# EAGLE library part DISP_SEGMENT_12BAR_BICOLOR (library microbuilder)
12-Bar Bi-Color LED Segment Displays: Row = Cathode 30.2 x 10.1mm Bi-Color 12 LED Bar Graph, 5.0 x 1.74mm Square LEDs - BL-AR12Z3010
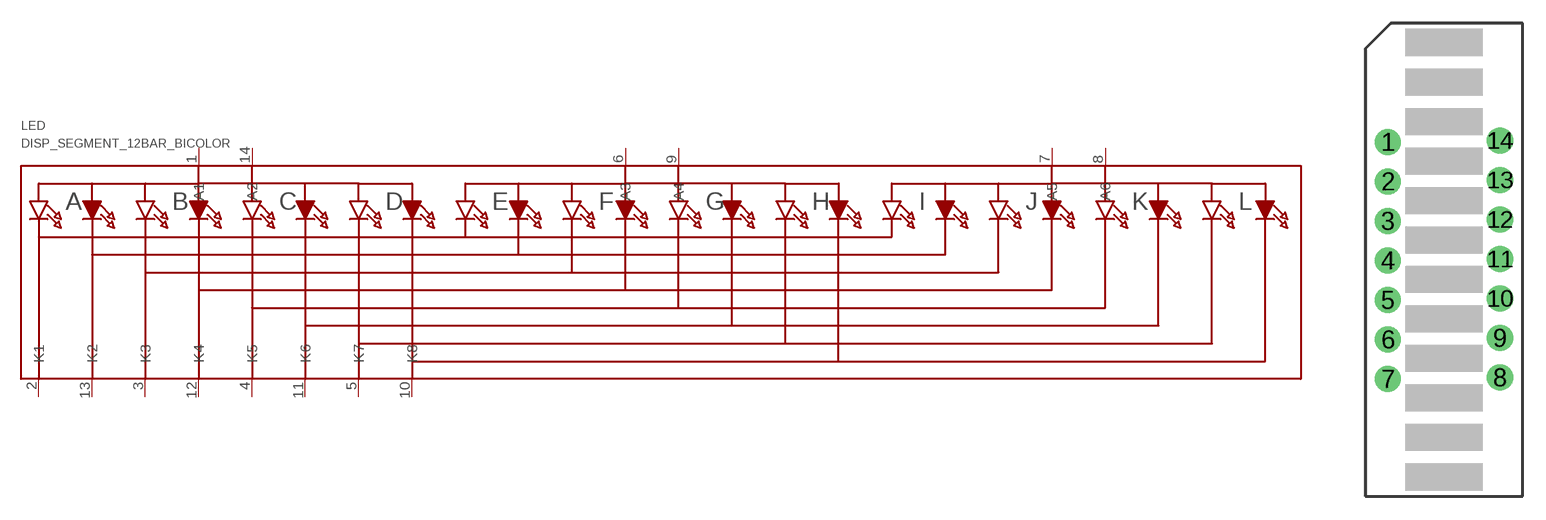
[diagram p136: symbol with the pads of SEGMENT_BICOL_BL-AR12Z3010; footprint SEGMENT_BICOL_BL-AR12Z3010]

Designator prefix LED

## DISP_SEGMENT_12BAR_BICOLORAR12Z3010  [SEGMENT_BICOL_BL-AR12Z3010]
1  A1
2  K1
3  K3
4  K5
5  K7
6  A3
7  A5
8  A6
9  A4
10  K8
11  K6
12  K4
13  K2
14  A2

## Footprint SEGMENT_BICOL_BL-AR12Z3010 (pad centres in mm)
Souce: http://www.betlux.com/product/LED_light_bar/BL-AR12B3010xx.PDF
drill 0.8 pad 1.676: 1 -3.6,7.57; 2 -3.6,5.03; 3 -3.6,2.49; 4 -3.6,-0.05; 5 -3.6,-2.59; 6 -3.6,-5.13; 7 -3.6,-7.67; 8 3.6,-7.57; 9 3.6,-5.03; 10 3.6,-2.49; 11 3.6,0.05; 12 3.6,2.59; 13 3.6,5.13; 14 3.6,7.67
